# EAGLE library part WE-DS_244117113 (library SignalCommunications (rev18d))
WE-DS D-SUB-Filter Connectors Bent 90° Characteristics Standard type filtered with 1000 pF High attenuation of more than 40 dB @ 180 MHz Low size: 6.3 mm Rated voltage: 125 VDC Rated current @ 20 ºC: 5 A Withstand voltage: 250 VRMS Insulation resistance: min. 1000 MΩ Operating temperature: –55 ºC to +125 ºC Applications Filtering of interfaces External connection to -printer -sensor -display Details see: http://katalog.we-online.de/en/pbs/D-SUB-Filter Bent 90° Created on 2015-05-04 2015 (C) Wurth Elektronik
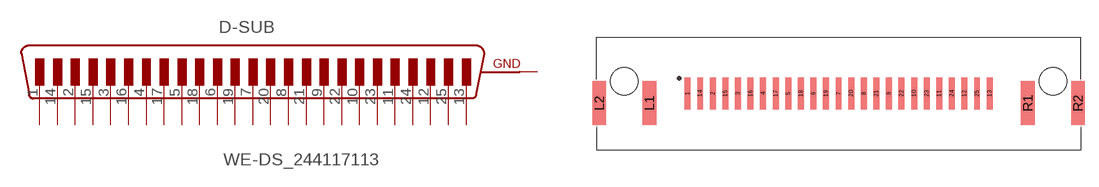
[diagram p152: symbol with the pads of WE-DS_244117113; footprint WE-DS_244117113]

Designator prefix D-SUB

## WE-DS_244117113 (WE-NUMBER: 244117113/25pins_male)  [WE-DS_244117113]
1  1  pas
2  2  pas
3  3  pas
4  4  pas
5  5  pas
6  6  pas
7  7  pas
8  8  pas
9  9  pas
10  10  pas
11  11  pas
12  12  pas
13  13  pas
14  14  pas
15  15  pas
16  16  pas
17  17  pas
18  18  pas
19  19  pas
20  20  pas
21  21  pas
22  22  pas
23  23  pas
24  24  pas
25  25  pas
L1  GND  pwr
L2  GND  pwr
R1  GND  pwr
R2  GND  pwr

## Footprint WE-DS_244117113 (pad centres in mm)
smd 0.65 x 3.5: 1 -16.56,0.02; 2 -13.8,0.02; 3 -11.04,0.02; 4 -8.28,0.02; 5 -5.52,0.02; 6 -2.76,0.02; 7 0,0.02; 8 2.76,0.02; 9 5.52,0.02; 10 8.28,0.02; 11 11.04,0.02; 12 13.8,0.02; 13 16.56,0.02; 14 -15.18,0.02; 15 -12.42,0.02; 16 -9.66,0.02; 17 -6.9,0.02; 18 -4.14,0.02; 19 -1.38,0.02; 20 1.38,0.02; 21 4.14,0.02; 22 6.9,0.02; 23 9.66,0.02; 24 12.42,0.02; 25 15.18,0.02
smd 1.5 x 4.8: L1 -20.75,-1.05; L2 -26.25,-1.05; R1 20.75,-1.05; R2 26.25,-1.05
hole 3 at -23.5,1.35
hole 3 at 23.5,1.35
